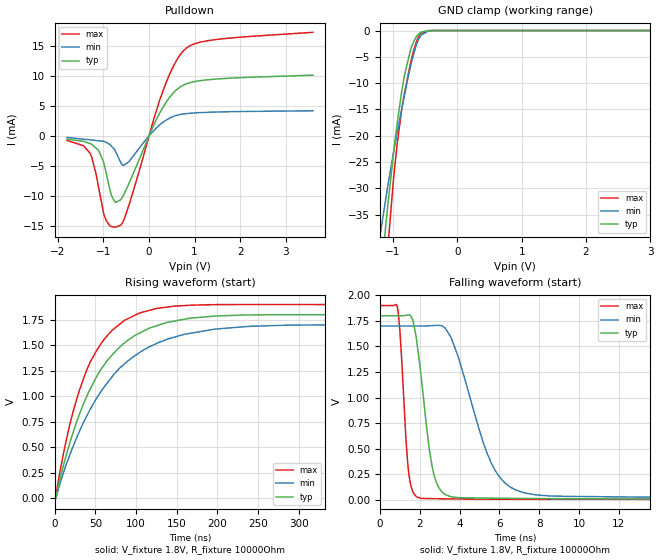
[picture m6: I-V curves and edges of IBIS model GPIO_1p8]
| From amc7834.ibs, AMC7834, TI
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|   Model
[Model]   GPIO_1p8
Model_type   I/O_open_drain
Polarity   Non-Inverting
Enable   Active-Low
Vinl = 0.54
Vinh = 1.26
Vmeas = 0.9
Vref = 1.8
Cref = 1pF
Rref = 10000
|   typ   min   max
C_comp   2.622pF   2.415pF   2.744pF
[Voltage Range]   1.8   1.7   1.9
[Temperature Range]   27   125   -40
[Pullup Reference]   1.8   1.7   1.9
[Pulldown Reference]   0   0   0
[Power Clamp Reference]   1.8   1.7   1.9
[GND Clamp Reference]   0   0   0
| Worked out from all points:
|   slope of the pulldown table from 0 to 0.27 V, typ, clamps not added: 62.9 ohm
|   GND clamp passes 1 mA (typ) near -0.62 V on its own axis
|   falling waveform, V_fixture 1.8V, R_fixture 10000Ohm: 20-80 % time 666ps typ, 1.62ns min, 339ps max; typ from 1.8 V to 0.01 V
|   rising waveform, V_fixture 1.8V, R_fixture 10000Ohm: 20-80 % time 62.6ns typ, 77.4ns min, 47.9ns max; typ from 0.01 V to 1.8 V
[Pulldown]
|   Voltage   I(typ)   I(min)   I(max)
-1.8V     -532.9uA   -264.1uA   -765.4uA
-1.298V   -1.279mA   -665.3uA   -2.861mA
-1.115V   -2.355mA   -811.5uA   -8.294mA
-936.4mV  -6.365mA   -1.103mA   -14.18mA
-822.6mV  -10.02mA   -1.74mA    -15.18mA
-736.2mV  -11.14mA   -2.577mA   -15.25mA
-622.8mV  -10.67mA   -4.416mA   -14.92mA
-444.6mV  -8.03mA    -4.334mA   -11.66mA
311.4mV   4.841mA    2.298mA    7.616mA
765mV     8.518mA    3.67mA     14.29mA
1.37V     9.427mA    3.96mA     15.99mA
3.6V      10.14mA    4.192mA    17.3mA
[GND Clamp]
|   Voltage   I(typ)   I(min)   I(max)
-1.8V     -130.2mA   -94.22mA   -169.2mA
-1.19V    -47mA      -38.28mA   -59.46mA
-1.093V   -34.91mA   -30.6mA    -43.38mA
-1.082V   -33.64mA   -29.79mA   -41.78mA
-995.4mV  -23.92mA   -23.57mA   -29.03mA
-938.3mV  -18.13mA   -19.77mA   -22.17mA
-822.6mV  -8.671mA   -12.49mA   -12.11mA
-709.2mV  -3.07mA    -5.994mA   -5.312mA
-633.6mV  -1.136mA   -2.723mA   -2.086mA
-563.4mV  -303.7uA   -885uA     -525.4uA
-347.4mV  -830.1nA   -8.806uA   -432.7nA
3.6V      0A         0A         0A
[POWER Clamp]
|   Voltage   I(typ)   I(min)   I(max)
-3.3V     0A         0A         0A
0V        0A         0A         0A
6.6V      0A         0A         0A
[Ramp]
R_load = 10000
|   typ   min   max
dV/dt_r   1.07414/6.24742e-08   1.009/7.74797e-08   1.13593/4.79234e-08
dV/dt_f   1.07413/6.65822e-10   1.009/1.6221e-09   1.13592/3.39461e-10
[Falling Waveform]
V_fixture = 1.8V
V_fixture_min = 1.7V
V_fixture_max = 1.9V
R_fixture = 10000Ohm
C_fixture = 0F
|   Time   V(typ)   V(min)   V(max)
0s        1.8V       1.7V       1.9V
870.8ps   1.8V       1.7V       1.889V
1.469ns   1.808V     1.7V       228.4mV
1.814ns   1.599V     1.7V       37.1mV
2.28ns    822.4mV    1.701V     14.69mV
2.698ns   258.4mV    1.705V     13.37mV
3.29ns    52.49mV    1.676V     11.66mV
5.914ns   17.68mV    249.5mV    7.888mV
9.261ns   12.67mV    36.25mV    6.98mV
500ns     9.822mV    18.68mV    6.773mV
[Rising Waveform]
V_fixture = 1.8V
V_fixture_min = 1.7V
V_fixture_max = 1.9V
R_fixture = 10000Ohm
C_fixture = 0F
|   Time   V(typ)   V(min)   V(max)
0s        9.822mV    18.68mV    6.773mV
1.98ns    33.34mV    15.81mV    57.08mV
12.1ns    367.5mV    286.6mV    495.3mV
21.48ns   619.9mV    489.9mV    817.8mV
42.87ns   1.06V      862.9mV    1.324V
69.97ns   1.401V     1.187V     1.644V
103.9ns   1.619V     1.428V     1.817V
140.4ns   1.729V     1.566V     1.878V
196.4ns   1.787V     1.659V     1.9V
500ns     1.8V       1.7V       1.9V
